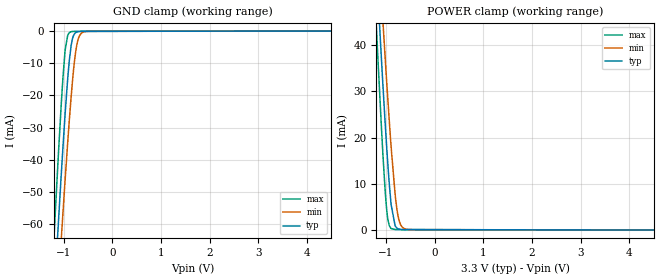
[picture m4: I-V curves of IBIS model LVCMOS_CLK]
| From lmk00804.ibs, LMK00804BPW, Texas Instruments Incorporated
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|   Model LVCMOS_CLK
[Model]   LVCMOS_CLK
Model_type   Input
Vinl = 1.3
Vinh = 2.0
|   typ   min   max
|   (nom PVT)   (fast PVT)   (slow PVT)
C_comp   0.302p   0.289p   0.313p
[Voltage Range]   3.3   3.135   3.465
[Temperature Range]   45   125   -40
[Power Clamp Reference]   3.3   3.135   3.465
[GND Clamp Reference]   0   0   0
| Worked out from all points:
|   GND clamp passes 1 mA (typ) near -0.78 V on its own axis
|   POWER clamp passes 1 mA (typ) near -0.82 V on its own axis
[GND Clamp]
|   Voltage   I(typ)   I(min)   I(max)
-3.3V     -686.4mA   -656mA     -728.4mA
-1.191V   -82.12mA   -99.87mA   -62.66mA
-1.102V   -58.61mA   -77.95mA   -37.27mA
-1.033V   -41.09mA   -61.34mA   -19.25mA
-963.6mV  -24.81mA   -45.34mA   -5.502mA
-914.1mV  -14.64mA   -34.47mA   -1.251mA
-844.8mV  -4.514mA   -20.55mA   -192.9uA
-775.5mV  -869.2uA   -9.382mA   -91.41uA
-716.1mV  -231.6uA   -3.488mA   -83.38uA
-656.7mV  -101.1uA   -1.066mA   -81.73uA
-557.7mV  -77.58uA   -169.1uA   -79.73uA
6.6V      0A         0A         0A
[POWER Clamp]
|   Voltage   I(typ)   I(min)   I(max)
-3.3V     501.3mA    474.5mA    538.8mA
-1.191V   55.5mA     67.62mA    42.21mA
-1.171V   51.63mA    64.05mA    37.96mA
-1.092V   36.48mA    49.98mA    21.61mA
-1.063V   31mA       44.82mA    15.96mA
-1.013V   22.25mA    36.4mA     7.713mA
-973.5mV  15.76mA    29.88mA    3.095mA
-894.3mV  5.386mA    17.76mA    304.8uA
-815.1mV  973.9uA    7.87mA     91.45uA
-755.7mV  272.5uA    3.151mA    84uA
-597.3mV  78.51uA    191uA      80.51uA
6.6V      0A         0A         0A
